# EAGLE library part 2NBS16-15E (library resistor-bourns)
BOURNS RESISTOR NETWORK
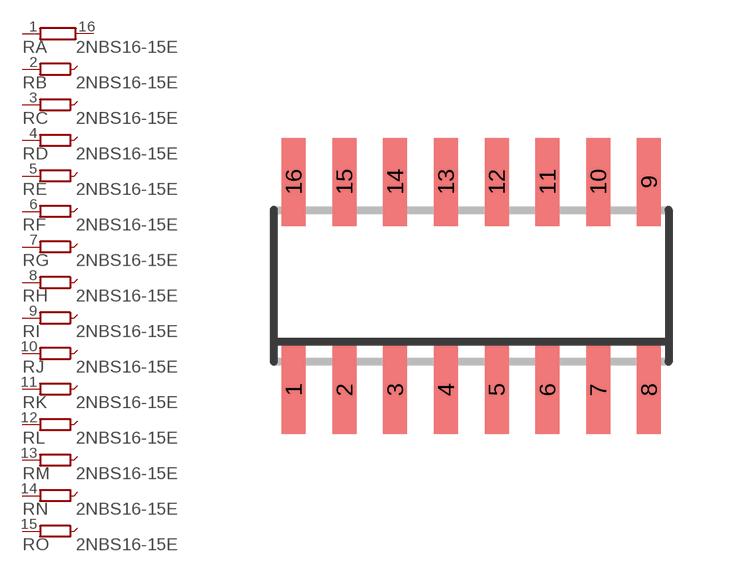
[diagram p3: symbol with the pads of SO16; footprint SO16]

Designator prefix R; gates A=R1NV B=R1NVXX C=R1NVXX D=R1NVXX E=R1NVXX F=R1NVXX G=R1NVXX H=R1NVXX I=R1NVXX J=R1NVXX K=R1NVXX L=R1NVXX M=R1NVXX N=R1NVXX O=R1NVXX

## 2NBS16-15E (OC_FARNELL: unknown; OC_NEWARK: unknown)  [SO16]
1  A:1  pas
2  B:1  pas
3  C:1  pas
4  D:1  pas
5  E:1  pas
6  F:1  pas
7  G:1  pas
8  H:1  pas
9  I:1  pas
10  J:1  pas
11  K:1  pas
12  L:1  pas
13  M:1  pas
14  N:1  pas
15  O:1  pas
16  A:2  pas

## Footprint SO16 (pad centres in mm)
BOURNS RESISTOR NETWORK
smd 0.6 x 2.2: 1 -4.445,-2.6; 2 -3.175,-2.6; 3 -1.905,-2.6; 4 -0.635,-2.6; 5 0.635,-2.6; 6 1.905,-2.6; 7 3.175,-2.6; 8 4.445,-2.6; 9 4.445,2.6; 10 3.175,2.6; 11 1.905,2.6; 12 0.635,2.6; 13 -0.635,2.6; 14 -1.905,2.6; 15 -3.175,2.6; 16 -4.445,2.6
